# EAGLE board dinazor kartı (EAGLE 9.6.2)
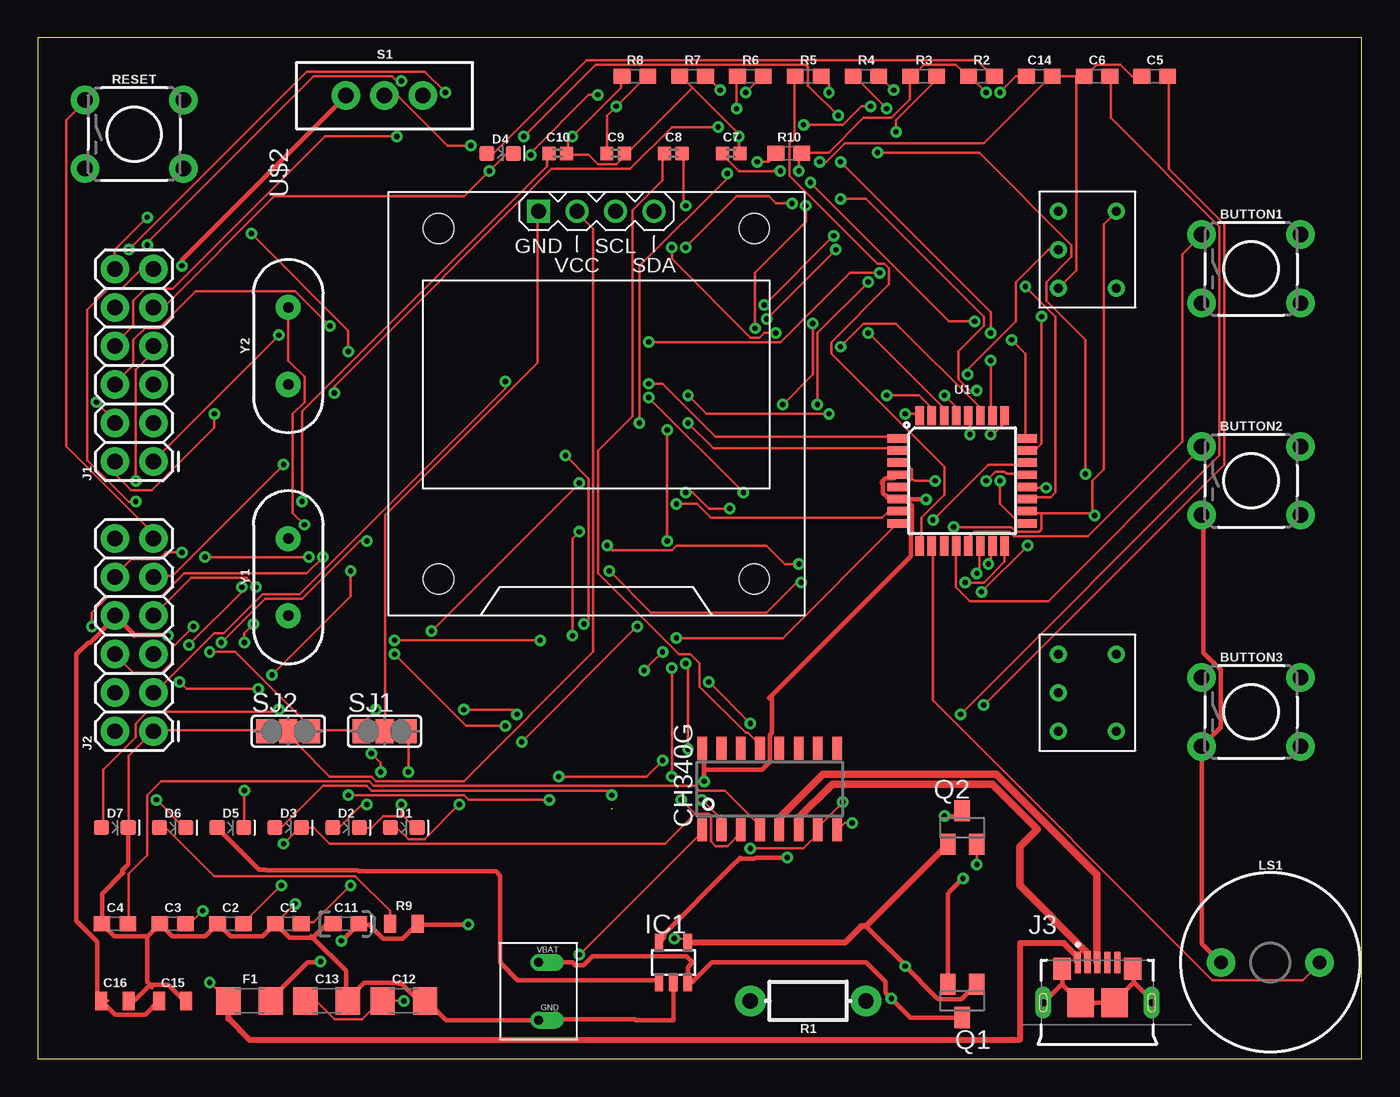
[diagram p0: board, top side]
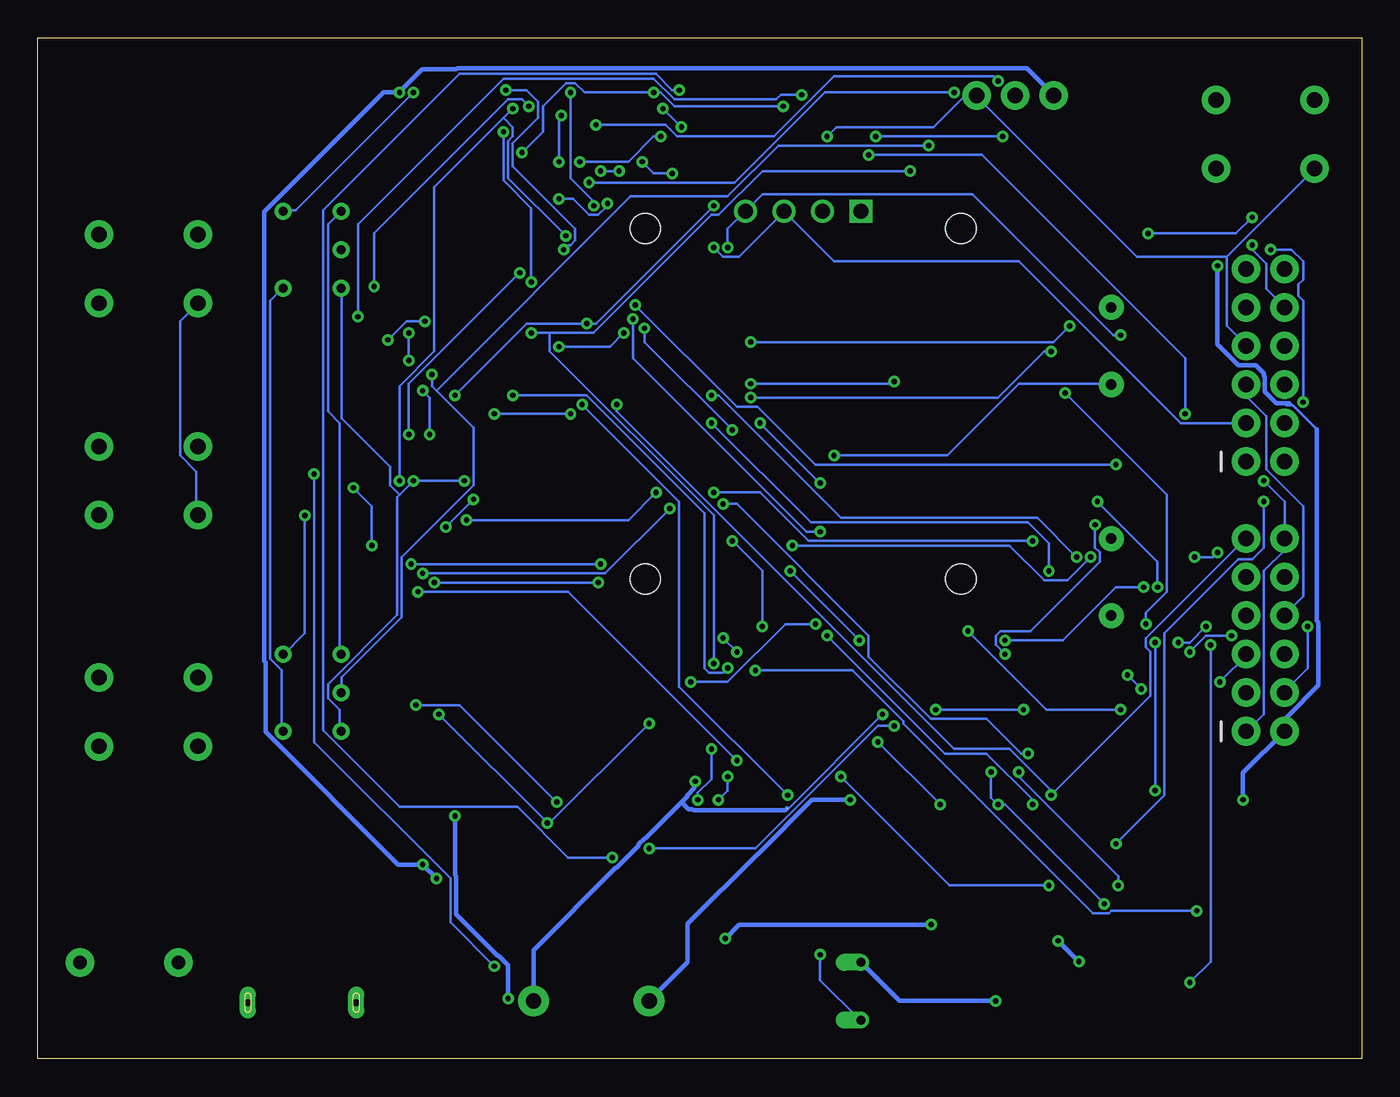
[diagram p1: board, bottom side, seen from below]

Size 87.3 x 67.3 mm. Coordinates in mm from the lower left corner, seen from the top.
Outline: 0,0 87.3,0 87.3,67.3 0,67.3 0,0
Copper layers (1*16): Top 0.035mm / dielectric 1.5mm / Bottom 0.035mm
Design rules "default": minimum track width 6mil, minimum drill 0.35mm, track to track 6mil, track to pad 6mil, pad to pad 6mil, via to via 6mil, smd to smd 6mil, copper to edge 40mil, drill to drill 6mil, minimum pad ring 10mil, minimum via ring 8mil, stop-mask expansion 4mil, vias tented up to drill 0mil, thermal gap 10mil

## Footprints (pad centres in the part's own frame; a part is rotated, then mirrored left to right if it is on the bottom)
TACTILE_SWITCH_PTH_6.0MM = drill 1.016 pad 1.88: 1 -3.251,2.261; 2 3.251,2.261; 3 -3.251,-2.261; 4 3.251,-2.261
0603 = smd 1.1 x 1: 1 -0.85,0; 2 0.85,0
0402 = smd 0.85 x 0.9: 1 -0.58,0; 2 0.58,0
0603-POLAR = smd 1.1 x 1: + 0.85,0; - -0.85,0
1206 = smd 1.6 x 1.8: 1 -1.4,0; 2 1.4,0
0805 = smd 0.8 x 1.2: 1 -0.9,0; 2 0.9,0
LED-0603 = smd 1 x 1: A -0.877,0; C 0.877,0
SOT23-5L = smd 0.55 x 1.2: 1 -0.95,-1.3; 2 0,-1.3; 3 0.95,-1.3; 4 0.95,1.3; 5 -0.95,1.3
2X6 = drill 1.016 pad 1.88: 1 0,0; 2 0,2.54; 3 2.54,0; 4 2.54,2.54; 5 5.08,0; 6 5.08,2.54; 7 7.62,0; 8 7.62,2.54; 9 10.16,0; 10 10.16,2.54; 11 12.7,0; 12 12.7,2.54
GCT_USB3075-30-A = smd 0.4 x 1.4: 1 0,0; 2 0.65,0; 3 1.3,0; 4 1.95,0; 5 2.6,0 | smd 1.15 x 1.45: S1 -1.02,-0.42; S2 3.62,-0.42 | smd 1.75 x 1.9: S3 0.175,-2.65; S4 2.425,-2.65 | drill 0.45 pad 1.05 long: S5 -2.275,-2.65; S6 4.875,-2.65
BUZZER-12MM-KIT = drill 0.9 pad 1.88: + 3.25,0; - -3.25,0
SOT23-BEC = smd 1 x 1.4: B -0.95,-1.1; C 0,1.1; E 0.95,-1.1
AXIAL-0.3-KIT = drill 1.016 pad 2.032: P$1 -3.81,0; P$2 3.81,0
SWITCH_SPDT_PTH_11.6X4.0MM = drill 1.016 pad 1.88: 1 0,2.54; 2 0,0; 3 0,-2.54
SJ_2 = smd 1.168 x 1.6: 1 -1.524,0; 2 0,0; 3 1.524,0
TQFP32-08 = smd 1.27 x 0.559: 1 -4.293,2.8; 2 -4.293,2; 3 -4.293,1.2; 4 -4.293,0.4; 5 -4.293,-0.4; 6 -4.293,-1.2; 7 -4.293,-2; 8 -4.293,-2.8; 17 4.293,-2.8; 18 4.293,-2; 19 4.293,-1.2; 20 4.293,-0.4; 21 4.293,0.4; 22 4.293,1.2; 23 4.293,2; 24 4.293,2.8 | smd 0.559 x 1.27: 9 -2.8,-4.293; 10 -2,-4.293; 11 -1.2,-4.293; 12 -0.4,-4.293; 13 0.4,-4.293; 14 1.2,-4.293; 15 2,-4.293; 16 2.8,-4.293; 25 2.8,4.293; 26 2,4.293; 27 1.2,4.293; 28 0.4,4.293; 29 -0.4,4.293; 30 -1.2,4.293; 31 -2,4.293; 32 -2.8,4.293
SOIC16 = smd 0.635 x 1.524: 1 -4.445,-2.695; 2 -3.175,-2.695; 3 -1.905,-2.695; 4 -0.635,-2.695; 5 0.635,-2.695; 6 1.905,-2.695; 7 3.175,-2.695; 8 4.445,-2.695; 9 4.445,2.695; 10 3.175,2.695; 11 1.905,2.695; 12 0.635,2.695; 13 -0.635,2.695; 14 -1.905,2.695; 15 -3.175,2.695; 16 -4.445,2.695
DISPLAY-OLED-128X64-I2C = drill 1 square: 1 -3.81,12.7 | drill 1: 2 -1.27,12.7; 3 1.27,12.7; 4 3.81,12.7 | hole 2: -10.414,11.557; 10.414,11.557; 10.414,-11.557; -10.414,-11.557
LİPOBATTERY = drill 0.6 offset: 1 -10.16,0; 2 -10.16,3.81
3.3V = drill 0.6: EN -6.35,0; GND -6.35,-2.54; IN -6.35,2.54; NC -2.54,-2.54; OUT -2.54,2.54
HC49US = drill 0.7 pad 1.651: 1 -2.54,0; 2 2.54,0

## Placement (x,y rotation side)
BUTTON1  MOMENTARY-SWITCH-SPST-PTH-6.0MM  [TACTILE_SWITCH_PTH_6.0MM]  80.01,52.07 0 top
BUTTON2  MOMENTARY-SWITCH-SPST-PTH-6.0MM  [TACTILE_SWITCH_PTH_6.0MM]  80.01,38.1 0 top
BUTTON3  MOMENTARY-SWITCH-SPST-PTH-6.0MM  [TACTILE_SWITCH_PTH_6.0MM]  80.01,22.86 0 top
C1  0.1uF  [0603]  16.51,8.89 0 top
C2  22pF  [0603]  12.7,8.89 0 top
C3  22pF  [0603]  8.89,8.89 0 top
C4  0.1uF  [0603]  5.08,8.89 0 top
C5  10pF  [0603]  73.66,64.77 0 top
C6  10pF  [0603]  69.85,64.77 0 top
C7  0.1uF  [0402]  45.72,59.69 0 top
C8  0.1uF  [0402]  41.91,59.69 0 top
C9  0.1uF  [0402]  38.1,59.69 0 top
C10  0.1uF  [0402]  34.29,59.69 0 top
C11  10uF  [0603-POLAR]  20.32,8.89 0 top
C12  4.7uF  [1206]  24.13,3.81 0 top
C13  4.7uF  [1206]  19.05,3.81 0 top
C14  0.1uF  [0603]  66.04,64.77 0 top
C15  2.2uF  [0805]  8.89,3.81 0 top
C16  10uF  [0805]  5.08,3.81 0 top
D1  BLUE  [LED-0603]  24.13,15.24 0 top
D2  BLUE  [LED-0603]  20.32,15.24 0 top
D3  GREEN  [LED-0603]  16.51,15.24 0 top
D4  Yellow  [LED-0603]  30.48,59.69 0 top
D5  GREEN  [LED-0603]  12.7,15.24 0 top
D6  GREEN  [LED-0603]  8.89,15.24 0 top
D7  RED  [LED-0603]  5.08,15.24 0 top
F1  6V/0.5A  [1206]  13.97,3.81 0 top
IC1  MCP73831  [SOT23-5L]  41.91,6.35 0 top
J1  2X6 FEMALE  [2X6]  7.62,39.37 90 top
J2  2X6 FEMALE  [2X6]  7.62,21.59 90 top
J3  USB3075-30-A  [GCT_USB3075-30-A]  68.58,6.35 0 top
LS1  BUZZER-PTH_KIT  [BUZZER-12MM-KIT]  81.28,6.35 0 top
Q1  BC327SMD  [SOT23-BEC]  60.96,3.81 180 top
Q2  BC327SMD  [SOT23-BEC]  60.96,15.24 0 top
R1  10k  [AXIAL-0.3-KIT]  50.8,3.81 180 top
R2  2.2k  [0603]  62.23,64.77 0 top
R3  2.2k  [0603]  58.42,64.77 0 top
R4  2.2k  [0603]  54.61,64.77 0 top
R5  2.2k  [0603]  50.8,64.77 0 top
R6  2.0k  [0603]  46.99,64.77 0 top
R7  2.0k  [0603]  43.18,64.77 0 top
R8  10k  [0603]  39.37,64.77 0 top
R9  0.22  [0805]  24.13,8.89 0 top
R10  2.2k  [0603]  49.53,59.69 0 top
RESET  MOMENTARY-SWITCH-SPST-PTH-6.0MM  [TACTILE_SWITCH_PTH_6.0MM]  6.35,60.96 0 top
S1  [SWITCH_SPDT_PTH_11.6X4.0MM]  22.86,63.5 270 top
SJ1  [SJ_2]  22.86,21.59 0 top
SJ2  [SJ_2]  16.51,21.59 0 top
U1  ATMEGA328P_TQFP  [TQFP32-08]  60.96,38.1 0 top
U$1  CH340G  [SOIC16]  48.26,17.78 0 top
U$2  DISPLAY-OLED-128X64-I2C  [DISPLAY-OLED-128X64-I2C]  36.83,43.18 0 top
U$3  LİPOBATTERY  [LİPOBATTERY]  43.18,2.54 0 top
U$4  3.3V  [3.3V]  73.66,53.34 0 top
U$5  3.3V  [3.3V]  73.66,24.13 0 top
Y1  16MHz  [HC49US]  16.51,31.75 90 top
Y2  16MHz  [HC49US]  16.51,46.99 90 top

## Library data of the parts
BUTTON1-BUTTON3 RESET = SparkFun-Switches; PROD_ID: SWCH-08441; SF_SKU: COM-00097
C1 C4 = SparkFun-Capacitors; PROD_ID: CAP-00810
C2 C3 = SparkFun-Capacitors; PROD_ID: CAP-07876
C5 C6 = SparkFun-Capacitors; PROD_ID: CAP-11812
C7-C10 = SparkFun-Capacitors; PROD_ID: CAP-12416
C11 = SparkFun-Capacitors; PROD_ID: CAP-13210
C12 C13 = SparkFun-Capacitors; PROD_ID: CAP-10300
C14 = SparkFun-Capacitors; PROD_ID: CAP-08604
C15 = SparkFun-Capacitors; PROD_ID: CAP-11624
C16 = SparkFun-Capacitors; PROD_ID: CAP-11330
D1 D2 = SparkFun-LED; PROD_ID: DIO-08575
D3 D5 D6 = SparkFun-LED; PROD_ID: DIO-00821
D4 = SparkFun-LED; PROD_ID: DIO-09003
D7 = SparkFun-LED; PROD_ID: DIO-00819
F1 = SparkFun-Fuses; PROD_ID: RES-08585
IC1 = microchip-update
J1 J2 = SparkFun-Connectors; PROD_ID: CONN-12423
J3 = USB3075-30-A; AVAILABILITY: In Stock; DESCRIPTION: USB - micro B USB 2.0 Receptacle Connector 5 Position Surface Mount, Right Angle; Through Hole, 2.35mm profile, 5 Pins, Horizontal, Bottom mount; MF: Global Connector Technology; MP: USB3075-30-A; PACKAGE: None; PRICE: None; PURCHASE-URL: https://pricing.snapeda.com/search/part/USB3075-30-A/?ref=eda
LS1 = SparkFun-Electromechanical; PROD_ID: COMP-08253; SF_SKU: COM-07950
Q1 Q2 = transistor-pnp
R1 = SparkFun-Resistors; PROD_ID: RES-09435
R2-R5 R10 = SparkFun-Resistors; PROD_ID: RES-08272
R6 R7 = SparkFun-Resistors; PROD_ID: RES-08296
R8 = SparkFun-Resistors; PROD_ID: RES-00824
R9 = SparkFun-Resistors; PROD_ID: RES-09883
S1 = SparkFun-Switches; PROD_ID: SWCH-08261; SF_SKU: COM-00102
SJ1 SJ2 = jumper
U1 = SparkFun-IC-Microcontroller; PROD_ID: IC-09069
U$1 = usb-serial
U$2 = diy-modules
U$3-U$5 = untitled
Y1 Y2 = SparkFun-Clocks; PROD_ID: XTAL-08181; SF_ID: COM-00536

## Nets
A0: J1.2 U1.23
A1: J1.4 U1.24
A2: J1.6 U1.25
A3: J1.8 U1.26
A4/SDA: J1.1 U1.27 U$2.4
A5/SCL: J1.3 U1.28 U$2.3
A6: J1.10 U1.19
A7: J1.12 U1.22
BUTTON1: BUTTON1.1 U1.13
BUTTON2: BUTTON2.1 U1.12
BUTTON3: U1.11
BUZZER: LS1.+ U1.10
D0/RX: D4.C J1.9 U1.30 U$1.2
D1/TX: D3.C J1.11 U1.31 U$1.3
D2: J2.4 U1.32
D3: J2.3 U1.1
D4: J2.5 U1.2
D10/SS: J2.6 U1.14
D11/MOSI: J2.10 U1.15
D12/MISO: J2.7 U1.16
D13/SCK: J2.9 R4.1 U1.17
D+: J3.3 U$1.5
D-: J3.2 U$1.6
GND: C1.1 C2.1 C3.1 C4.1 C5.1 C6.1 C7.2 C9.2 C10.2 C11.- C12.2 C13.2 C14.2 C15.2 C16.2 D1.C D2.C D7.C IC1.2 J1.7 J2.1 J2.12 R7.1 R8.1 RESET.3 S1.1 SJ1.3 SJ2.1 U1.3 U1.5 U1.21 U$1.1 U$3.1 U$4.GND U$5.GND
LED: R5.1 U1.9
N$1: D3.A R3.2
N$2: C1.2 U1.20
N$3: C4.2 U$1.4
N$4: C2.2 U1.7
N$5: C3.2 U1.8
N$6: C6.2 U$1.8 Y2.1
N$7: C5.2 U$1.7 Y2.2
N$8: D4.A R2.2
N$9: C8.1 U$1.13
N$10: SJ1.2 U$2.1
N$11: SJ2.2 U$2.2
N$12: BUTTON3.1
N$13: D2.A R4.2
N$14: D1.A R5.2
N$15: J3.S1 J3.S2 J3.S3 J3.S4 J3.S5 J3.S6
N$16: J3.5
N$17: BUTTON1.3 BUTTON2.3 BUTTON3.3 LS1.-
N$18: C10.1 F1.1 J3.1
N$19: D5.C R6.1
N$20: D5.A IC1.1
N$21: D6.A R9.1
N$22: IC1.5 R7.2
N$23: U$4.IN U$5.IN
N$24: S1.2 U$4.EN U$5.EN
N$26: U$4.NC U$5.NC
N$31: D7.A R10.1
RESET: C8.2 J2.11 R1.P$2 RESET.1 U1.29
V_BATT: C12.1 C13.1 IC1.3 Q1.C Q2.C U$3.2
VCC: C7.1 C15.1 C16.1 J1.5 J2.8 R1.P$1 R2.1 R3.1 R10.2 SJ1.1 SJ2.3 U1.4 U1.6 U1.18 U$1.16 U$4.OUT U$5.OUT
VIN: C14.1 D6.C J2.2 Q1.E Q2.E S1.3
VUSB: C9.1 C11.+ F1.2 IC1.4 Q1.B Q2.B R6.2 R8.2 R9.2

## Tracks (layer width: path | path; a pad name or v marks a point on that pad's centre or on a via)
A0  (via drill 0.35)
  Top 0.152: v66.19,48.92 66.19,40.54 65.89,40.23 65.28,40.23 U1.23 | v36.93,63.55 36.32,63.55 32.51,59.74 v32.51,59.59 | v11.63,42.52 11.63,41.6 7.52,37.49 6.15,37.49 5.08,38.56 J1.2
  Bottom 0.152: v66.19,48.92 66.19,55.02 56.59,64.62 46.69,64.62 45.31,63.25 38.61,63.25 38.3,63.55 v36.93,63.55 | v32.51,59.59 25.04,59.59 11.63,46.18 v11.63,42.52
A1  (via drill 0.35)
  Top 0.152: v64.21,47.4 65.13,46.48 65.13,41 U1.24 | v61.77,48.62 60.1,48.62 v50.95,57.76 | v26.87,63.7 25.5,65.08 17.73,65.08 v5.99,53.34 | v3.86,43.28 5.08,42.06 J1.4
  Bottom 0.152: v64.21,47.4 62.99,48.62 v61.77,48.62 | v50.95,57.76 41.35,57.76 35.41,63.7 v26.87,63.7 | v5.99,53.34 4.62,53.34 3.86,52.58 3.86,51.36 4.17,51.05 4.17,50.29 3.86,49.99 v3.86,43.28
A2  (via drill 0.35)
  Top 0.152: v62.84,41.15 62.99,41.15 63.75,41.91 63.75,42.37 U1.25 | v55.52,51.82 53.54,51.82 48.97,47.24 v40.28,47.24 | v19.25,48.31 16.97,50.6 10.41,50.6 7.98,48.16 7.06,48.16 6.3,47.4 6.3,45.72 5.08,44.5 J1.6
  Bottom 0.152: v62.84,41.15 62.84,44.5 v55.52,51.82 | v40.28,47.24 20.32,47.24 v19.25,48.31
A3  (via drill 0.35)
  Top 0.152: v62.84,46.02 62.84,42.52 U1.26 | v62.84,47.85 62.84,49.23 v52.93,59.13 | v52.78,62.18 50.8,64.16 50.8,65.38 50.65,65.53 36.78,65.53 v32.05,60.81 | v23.67,60.81 18.95,60.81 8.89,50.75 7.06,50.75 6.3,49.99 6.3,48.31 5.08,47.09 J1.8
  Bottom 0.152: v62.84,47.85 v62.84,46.02 | v52.93,59.13 52.93,62.03 v52.78,62.18 | v23.67,60.81 v32.05,60.81
A4/SDA  (via drill 0.35)
  Top 0.152: v52.93,46.94 54.46,48.46 56.59,48.46 62.08,42.98 62.08,42.52 U1.27 | v48.67,47.85 47.9,47.85 47.6,47.55 46.99,47.55 41.81,52.73 v41.81,53.49 | v15.9,47.7 7.67,39.47 J1.1
  Bottom 0.152: v52.93,46.94 49.58,46.94 v48.67,47.85 | v41.81,53.49 41.81,54.71 U$2.4 39.52,57 25.65,57 16.36,47.7 v15.9,47.7
A5/SCL  (via drill 0.35)
  Top 0.152: v61.47,41.15 61.47,42.37 U1.28 | v61.93,44.04 61.47,44.04 60.71,44.81 60.71,46.63 62.38,48.31 62.38,48.92 54.61,56.69 v52.93,56.69 | v49.73,56.39 48.67,56.39 48.21,56.84 46.08,56.84 v42.72,53.49
  Bottom 0.152: v61.47,41.15 61.47,43.59 v61.93,44.04 | v52.93,56.69 52.02,56.69 50.95,55.63 50.34,55.63 49.73,56.24 v49.73,56.39 | v42.72,53.49 42.11,52.88 41.05,52.88 38.15,55.78 U$2.3 34.8,52.58 22.61,52.58 11.94,41.91 J1.3
A6  (via drill 0.35)
  Top 0.152: v65.13,50.9 67.11,48.92 67.11,37.34 66.8,37.03 65.28,37.03 U1.19 | v54.92,62.79 54.3,62.79 53.09,61.57 v50.5,61.57 | v23.98,64.47 23.67,64.47 23.37,64.77 18.19,64.77 7.21,53.8 v7.21,53.65
  Bottom 0.152: v65.13,50.9 65.13,54.41 56.29,63.25 55.37,63.25 v54.92,62.79 | v50.5,61.57 45.92,61.57 45.16,60.81 38.76,60.81 34.8,64.77 24.28,64.77 v23.98,64.47 | v7.21,53.65 7.21,53.34 6.3,52.43 6.3,50.75 J1.10
A7  (via drill 0.35)
  Top 0.152: v59.03,35.51 62.69,39.17 65.13,39.17 U1.22 | v40.28,43.59 v46.53,37.34 | v20.47,46.63 20.47,48.01 v14.07,54.41 | v7.21,55.47 5.08,53.34 J1.12
  Bottom 0.152: v59.03,35.51 48.36,35.51 v46.53,37.34 | v40.28,43.59 23.98,43.59 20.93,46.63 v20.47,46.63 | v14.07,54.41 8.28,54.41 v7.21,55.47
BUTTON1
  Top 0.152: U1.13 61.47,33.83 61.47,34.44 61.77,34.75 64.06,34.75 64.36,34.44 69.24,34.44 75.49,40.69 75.49,53.03 76.71,54.25 BUTTON1.1
BUTTON2
  Top 0.152: U1.12 60.55,33.68 60.55,31.09 61.47,30.18 66.65,30.18 76.71,40.23 BUTTON2.1
BUZZER
  Top 0.152: U1.10 59.03,33.68 59.03,23.62 77.47,5.18 83.41,5.18 84.48,6.25 LS1.+
D0/RX  (via drill 0.35)
  Top 0.152: J1.9 8.28,49.53 15.6,56.84 28.09,56.84 v29.77,58.52 30.84,59.59 31.29,59.59 D4.C | v54.76,47.85 59.64,42.98 59.64,42.52 U1.30 | v43.79,17.07 45.01,15.85 45.01,15.09 U$1.2 | v42.88,20.42 42.88,25.91 v42.72,26.06
  Bottom 0.152: 53.54,47.85 50.65,47.85 42.88,55.63 42.42,55.63 39.52,58.52 v29.77,58.52 | 53.54,47.85 v54.76,47.85 | v43.79,17.07 43.79,17.53 42.88,18.44 v42.88,20.42 | v42.72,26.06 42.72,35.81 53.54,46.63 53.54,47.85
D1/TX  (via drill 0.35)
  Top 0.152: 43.33,16.15 41.35,14.17 19.25,14.17 18.19,15.24 D3.C 17.27,15.24 v16.21,14.17 | 43.33,16.15 44.25,16.15 44.4,16 44.4,14.33 44.7,14.02 45.47,14.02 46.38,14.94 U$1.3 | v55.98,43.74 58.12,43.74 58.88,42.98 58.88,42.52 U1.31 | v41.81,18.59 v41.81,25.76 | 43.33,16.15 v42.42,17.07 | v6.45,36.73 5.99,36.73 3.25,39.47 3.25,49.38 4.62,50.75 5.54,50.75 6.76,51.97 7.52,51.97 J1.11
  Bottom 0.152: v55.98,43.74 51.11,43.74 43.33,35.97 43.33,25.76 43.03,25.45 42.11,25.45 v41.81,25.76 | v41.81,18.59 41.81,17.68 v42.42,17.07 | v6.45,36.73 6.45,33.68 7.21,32.92 8.13,32.92 13,28.04 13,17.37 v16.21,14.17
D2  (via drill 0.35)
  Top 0.152: v57.2,42.52 58.12,42.52 U1.32 | v52.17,42.52 44.09,42.52 v42.88,43.74 | v18.8,33.07 17.73,32 9.65,32 8.13,30.48 4.62,30.48 3.56,29.41 v3.56,28.5
  Bottom 0.152: v52.17,42.52 v57.2,42.52 | v42.88,43.74 42.42,43.74 34.34,35.66 21.39,35.66 v18.8,33.07 | v3.56,28.5 3.56,25.76 5.08,24.23 J2.4
D3  (via drill 0.35)
  Top 0.152: v40.28,44.5 41.2,44.5 44.7,41 56.59,41 U1.1 | v30.84,44.65 30.84,44.2 17.27,30.63 14.83,30.63 12.24,28.04 11.63,28.04 7.67,24.08 J2.3
  Bottom 0.152: v40.28,44.5 30.99,44.5 v30.84,44.65
D4  (via drill 0.35)
  Top 0.152: v42.88,41.91 44.55,40.23 56.59,40.23 U1.2 | v20.62,32.16 20.62,30.48 v15.44,25.3 | v14.53,24.38 9.8,24.38 v9.35,24.84
  Bottom 0.152: v42.88,41.91 36.32,35.36 22,35.36 20.62,33.98 v20.62,32.16 | v14.53,24.38 v15.44,25.3 | v9.35,24.84 7.52,26.67 J2.5
D10/SS  (via drill 0.35)
  Top 0.152: v61.93,32 62.08,32.16 62.08,33.68 U1.14 | v45.62,36.27 44.25,36.27 43.18,37.34 v42.72,37.34 | v21.69,34.14 21.23,34.14 17.42,30.33 14.99,30.33 v12.09,27.43 | v10.26,28.5 8.89,27.13 8.89,26.21 8.13,25.45 6.3,25.45 J2.6
  Bottom 0.152: v61.93,32 49.89,32 v45.62,36.27 | v42.72,37.34 39.68,37.34 36.47,34.14 v21.69,34.14 | v12.09,27.43 11.33,27.43 v10.26,28.5
D11/MOSI  (via drill 0.35)
  Top 0.152: v62.69,32.61 62.84,32.77 62.84,33.68 U1.15 | v50.19,32.61 49.28,32.61 48.06,33.83 42.11,33.83 41.81,33.53 37.85,33.53 v37.54,33.83 | v11.02,33.07 v17.88,33.07 | v9.5,33.38 8.43,33.38 7.98,32.92 6.15,32.92 5.08,31.85 J2.10
  Bottom 0.152: v50.19,32.61 v62.69,32.61 | v37.54,33.83 23.22,33.83 20.93,31.55 19.41,31.55 v17.88,33.07 | v11.02,33.07 9.8,33.07 v9.5,33.38
D12/MISO  (via drill 0.35)
  Top 0.152: v61.16,31.39 62.38,31.39 63.75,32.77 63.75,33.68 U1.16 | v50.34,31.39 50.04,31.39 48.06,29.41 40.44,29.41 v37.69,32.16 | v23.52,27.58 v33.12,27.58 | v14.38,31.09 13.77,31.7 10.11,31.7 J2.7
  Bottom 0.152: v50.34,31.39 v61.16,31.39 | v33.12,27.58 v37.69,32.16 | v23.52,27.58 19.71,27.58 16.21,31.09 v14.38,31.09
D13/SCK  (via drill 0.35)
  Top 0.152: v55.98,62.64 53.85,64.77 R4.1 | v63.45,38.1 63.45,36.58 64.67,35.36 65.13,35.36 U1.17 | v16.21,39.17 8.89,31.85 7.67,31.85 J2.9 | v52.48,54.25 v47.9,49.68
  Bottom 0.152: 56.59,62.03 61.16,57.45 61.16,46.63 63.45,44.35 v63.45,38.1 | 56.59,62.03 v55.98,62.64 | v16.21,39.17 36.02,39.17 39.83,42.98 41.2,42.98 v47.9,49.68 | v52.48,54.25 56.29,58.06 56.29,60.5 55.98,60.81 55.98,61.42 56.59,62.03
D+
  Top 0.152: 48.97,15.39 48.97,15.24 48.97,15.09 U$1.5 | 69.85,6.4 J3.3
  Top 0.508: J3.3 69.85,6.38 69.85,12.12 63.21,18.76 51.78,18.76 51.03,18.01 50.8,17.78 48.97,15.95 48.97,15.24
D-
  Top 0.152: 50.19,15.39 50.19,15.09 U$1.6 | 69.09,6.4 J3.2
  Top 0.508: J3.2 69.23,6.97 64.77,11.43 64.77,13.97 65.92,15.12 62.94,18.1 52.39,18.1 50.17,15.88 U$1.6
GND  (via drill 0.35)
  Top 0.152: SJ2.1 14.99,21.64 7.67,21.64 J2.1 5.99,19.96 5.99,15.24 D7.C 5.84,15.24 | 41.81,4.57 41.81,5.03 IC1.2 | 39.83,2.59 39.37,2.59 | 33.12,2.59 U$3.1 32.97,2.59 | v35.71,6.86 43.79,14.94 U$1.1 | 4.32,8.84 C4.1 4.32,8.99 | 7.98,8.84 C3.1 8.13,8.84 | 6.35,3.81 C16.2 | D2.C 22,15.24 22.76,16 23.98,16 | 23.98,16 24.13,16 24.89,15.24 D1.C | v24.43,18.9 24.43,21.49 SJ1.3 | 23.98,16 v23.98,16.76 | 11.94,8.84 C2.1 11.79,8.84 | 15.6,8.84 C1.1 | 19.05,8.84 19.41,8.84 C11.- | 15.75,8.84 C1.1 | 20.32,3.81 C13.2 20.47,3.81 | 25.04,3.81 25.4,3.81 C12.2 25.65,3.81 | 21.67,5 21.69,5.03 | v16.97,10.21 15.75,8.99 C1.1 | 26.8,2.67 26.87,2.59 | C6.1 68.48,64.77 | 68.48,64.77 C14.2 66.8,64.77 62.38,60.35 53.24,60.35 52.02,59.13 v51.56,59.13 | C5.1 72.14,64.77 71.37,65.53 69.85,65.53 69.09,64.77 C6.1 | 57.66,38.25 57.2,37.8 56.74,37.8 U1.5 | 57.66,38.25 57.66,38.86 57.35,39.17 56.74,39.17 U1.3 | v62.54,38.1 63.14,38.71 63.75,38.71 63.91,38.56 65.13,38.56 U1.21 | v59.18,38.1 57.81,38.1 57.66,38.25 | 68.48,64.77 68.48,51.97 U$4.GND | 68.94,64.77 C6.1 | 43.18,64.01 42.42,64.77 R7.1 | 43.18,64.01 46.23,60.96 v46.23,60.81 46.23,59.74 C7.2 | 38.76,59.59 38.15,58.98 36.93,58.98 36.32,59.59 34.95,59.59 C10.2 34.95,59.74 34.95,60.5 v35.26,60.81 38.46,64.01 38.46,64.77 R8.1 | 38.76,59.59 43.18,64.01 | 38.76,59.59 C9.2 | v6.45,38.1 6.45,45.41 7.52,46.48 7.52,46.94 J1.7
  Top 0.305: IC1.2 41.91,2.54 39.42,2.54 39.37,2.59 32.97,2.59 | U$3.1 26.92,2.54 26.8,2.67 25.65,3.81 25.4,3.81 | C12.2 25.1,3.81 23.98,4.93 | 23.82,5.03 23.88,5.03 23.98,4.93 | 23.98,4.93 23.74,4.93 23.66,5.01 21.8,5.01 21.79,5 21.67,5 21.51,5 20.32,3.81 | C13.2 20.32,3.94 20.32,5.79 18.14,7.98 | 18.03,8.08 18.14,7.98 | 18.14,7.98 19,8.84 19.05,8.84 | 18.14,7.98 16.61,7.98 15.75,8.84 | 15.6,8.84 14.83,8.08 12.7,8.08 11.94,8.84 | C2.1 11.04,8.08 8.85,8.08 C3.1 7.23,8.08 7.21,8.08 | 7.21,5.03 7.21,5.08 | 7.21,5.08 7.21,8.08 | 7.21,8.08 5.04,8.08 C4.1 4.23,10.88 5.56,12.22 | 5.56,12.22 5.61,12.27 | 5.56,12.22 5.56,12.42 5.96,12.81 D7.C | 7.21,5.08 7.42,4.88 | 7.42,4.88 7.52,4.78 | 7.52,4.78 7.52,4.72 | 7.42,4.88 8.59,4.88 9.65,3.81 C15.2 | 6.35,3.81 7.31,4.78 7.52,4.78
  Bottom 0.152: J2.1 7.52,21.64 6.45,22.71 6.45,32.16 5.08,33.53 J2.12 5.08,36.73 v6.45,38.1 | v35.71,6.86 35.71,5.18 33.12,2.59 U$3.1 | v24.43,18.9 24.43,17.22 v23.98,16.76 23.52,16.76 v16.97,10.21 | v59.18,38.1 v62.54,38.1 63.45,37.19 | 63.45,37.19 63.6,37.03 63.6,29.26 68.17,24.69 68.17,23.77 67.41,23.01 67.41,21.64 U$5.GND | 63.45,37.19 64.06,37.8 64.06,39.01 67.26,42.22 67.26,50.75 U$4.GND | 8.89,52.88 3.1,58.67 RESET.3 | 8.89,52.88 8.89,48.31 7.67,47.09 J1.7 | v35.26,60.81 34.65,61.42 28.25,61.42 26.26,63.4 25.5,63.4 S1.1 25.35,63.4 14.83,52.88 8.89,52.88 | v51.56,59.13 48.36,59.13 46.69,60.81 v46.23,60.81
LED
  Top 0.152: R5.1 49.89,64.77 49.89,60.66 49.58,60.35 49.58,58.22 55.37,52.43 55.83,52.43 56.13,52.12 56.13,51.05 52.32,47.24 52.32,46.48 59.79,39.01 59.79,37.19 58.27,35.66 58.27,33.83 U1.9
N$1  (via drill 0.35)
  Top 0.152: D3.A 16.05,15.24 18.8,17.98 21.69,17.98 22,17.68 37.54,17.68 v37.85,17.37 | v51.41,43.13 51.41,47.85 v54.76,51.21 | v56.59,61.11 56.59,61.87 59.18,64.47 59.18,64.77 R3.2
  Bottom 0.152: v37.85,17.37 45.01,24.54 45.01,36.73 v51.41,43.13 | v54.76,51.21 54.76,56.08 56.59,57.91 v56.59,61.11
N$2  (via drill 0.35)
  Top 0.152: v20.62,11.43 18.19,8.99 17.42,8.99 C1.2 | v34.34,18.59 40.13,18.59 v41.2,19.66 | v65.28,33.83 v62.23,30.79 | v66.5,37.64 65.28,37.64 U1.20
  Bottom 0.152: v20.62,11.43 27.18,11.43 v34.34,18.59 | v41.2,19.66 52.32,30.79 v62.23,30.79 | v65.28,33.83 65.28,36.42 v66.5,37.64
N$3
  Top 0.152: C4.2 5.99,8.99 5.99,12.19 7.21,13.41 7.21,17.37 8.13,18.29 21.84,18.29 22.15,17.98 43.33,17.98 43.64,17.68 45.31,17.68 47.6,15.39 47.6,15.09 U$1.4
N$4  (via drill 0.35)
  Top 0.152: v16.05,11.43 13.61,8.99 C2.2 | v22.61,18.9 22.61,19.51 v22,20.12 | v42.11,36.58 43.49,36.58 44.4,35.66 55.68,35.66 55.98,35.97 56.59,35.97 U1.7
  Bottom 0.152: v16.05,11.43 16.05,12.04 22.61,18.59 v22.61,18.9 | v22,20.12 22.45,20.12 24.74,22.4 28.4,22.4 32.51,26.52 32.51,27.89 41.2,36.58 v42.11,36.58
N$5  (via drill 0.35)
  Top 0.152: v10.87,9.75 10.11,8.99 9.8,8.99 C3.2 | v41.2,26.82 v39.98,25.6 | v42.11,27.74 49.12,27.74 56.59,35.2 U1.8
  Bottom 0.152: v10.87,9.75 16.51,9.75 16.66,9.6 17.73,9.6 30.23,22.1 30.23,22.25 33.58,25.6 v39.98,25.6 | v42.11,27.74 v41.2,26.82
N$6  (via drill 0.35)
  Top 0.152: v60.86,22.71 77.93,39.78 77.93,54.86 70.76,62.03 70.76,64.77 C6.2 | v53.7,15.54 53.24,15.54 52.78,15.09 U$1.8 | v34.8,39.78 36.32,38.25 36.32,28.96 v36.02,28.65 | v46.99,22.1 v44.25,24.84
  Bottom 0.152: v60.86,22.71 v53.7,15.54 53.54,15.54 v46.99,22.1 | v34.8,39.78 27.33,39.78 22.61,44.5 16.51,44.5 Y2.1 | v36.02,28.65 38,28.65 41.81,24.84 v44.25,24.84
N$7  (via drill 0.35)
  Top 0.152: v62.38,23.32 78.23,39.17 78.23,55.02 74.57,58.67 74.57,64.77 C5.2 | v53.09,16.92 51.56,15.39 51.56,15.09 U$1.7 51.56,14.94 50.5,13.87 v46.99,13.87 | Y2.2 16.51,46.02 17.58,44.96 17.58,43.28 16.82,42.52 16.82,35.97 v17.58,35.2 | v23.52,26.67 28.25,21.95 v30.84,21.95
  Bottom 0.152: v62.38,23.32 59.49,23.32 v53.09,16.92 | v17.58,35.2 17.58,33.68 17.27,33.38 17.27,32.77 21.84,28.19 23.82,28.19 24.13,27.89 24.13,27.28 v23.52,26.67 | v30.84,21.95 31.9,21.95 39.98,13.87 v46.99,13.87
N$8
  Top 0.152: D4.A 29.62,59.74 30.07,59.74 36.17,65.84 61.93,65.84 62.99,64.77 R2.2
N$9
  Top 0.152: C8.1 41.2,59.59 41.2,57.91 39.22,55.93 39.22,42.37 36.93,40.08 36.93,32 42.27,26.67 43.03,26.67 43.64,26.06 43.64,24.54 46.69,21.49 46.84,21.49 47.75,20.57 U$1.13
N$10
  Top 0.152: SJ1.2 22.91,21.64 22.91,35.81 32.97,45.87 32.97,55.78 U$2.1
N$11
  Top 0.152: SJ2.2 16.51,21.49 17.12,20.88 17.12,20.73 19.25,18.59 22,18.59 22.3,18.29 28.09,18.29 36.63,26.82 36.63,54.71 35.56,55.78 U$2.2
N$13  (via drill 0.35)
  Top 0.152: D2.A 19.86,15.24 21.39,16.76 v21.69,16.76 | v35.26,27.89 35.26,34.29 v35.71,34.75 | v52.63,53.34 v48.06,48.77 | v56.44,63.86 55.52,64.77 R4.2
  Bottom 0.152: v21.69,16.76 21.69,17.07 24.74,20.12 27.48,20.12 v35.26,27.89 | v35.71,34.75 36.63,34.75 48.06,46.18 v48.06,48.77 | v52.63,53.34 52.32,53.65 52.17,53.65 51.87,53.95 51.87,54.71 55.98,58.83 55.98,60.35 54.3,62.03 54.3,63.09 55.07,63.86 v56.44,63.86
N$14  (via drill 0.35)
  Top 0.152: D1.A 23.67,15.24 24.43,14.48 25.5,14.48 v27.79,16.76 | v39.52,28.5 v31.9,20.88 | v41.5,41.45 v41.5,34.14 | v47.3,48.16 47.3,51.82 50.65,55.17 v50.65,56.24 | v52.17,63.7 52.17,64.31 51.71,64.77 R5.2
  Bottom 0.152: v31.9,20.88 v27.79,16.76 | v39.52,28.5 39.52,32.16 v41.5,34.14 | v41.5,41.45 47.3,47.24 v47.3,48.16 | v50.65,56.24 50.65,56.54 52.17,58.06 v52.17,63.7
N$15
  Top 0.152: 67.56,4.88 67.56,5.03 | 67.56,5.79 J3.S1 | 68.63,3.81 J3.S3 68.78,3.66 | 72.29,5.79 J3.S2 | 73.35,3.81 J3.S6 | 71.07,3.81 J3.S4 70.92,3.66
  Top 0.305: 72.29,5.03 73.45,3.86 J3.S6 | 72.29,5.03 72.29,5.79 | 72.29,5.03 71.12,3.86 71.12,3.81 71.07,3.81 | J3.S4 J3.S3 67.56,4.89 | 67.56,4.89 67.56,5.03 67.56,5.79 | 67.56,4.89 67.5,4.89 J3.S5
N$17
  Top 0.152: 76.86,20.57 BUTTON3.3 76.86,20.73 | 77.93,6.4 LS1.- | 76.86,35.81 BUTTON2.3
  Top 0.305: 77.93,6.4 76.76,7.57 BUTTON3.3 76.76,20.62 78,21.87 78,25.64 | 77.93,25.76 78,25.68 78,25.64 | 78,25.64 76.86,26.78 76.86,26.82 76.86,35.81
  Bottom 0.152: BUTTON2.3 76.86,35.97 76.86,38.71 77.93,39.78 77.93,48.62 76.86,49.68 BUTTON1.3
N$18  (via drill 0.35)
  Top 0.152: v17.42,36.73 17.42,42.67 33.58,58.83 33.58,59.59 C10.1 | v13.46,31.09 13.46,30.79 v9.96,27.28 | v11.33,5.03 12.55,3.81 F1.1 12.7,3.81 | 68.48,6.71 68.48,6.4 J3.1
  Top 0.406: J3.1 68.49,6.44 68.49,6.8 67.67,7.62 64.77,7.62 64.77,1.27 64.72,1.22 13.97,1.22 12.57,2.62 F1.1
  Bottom 0.152: v17.42,36.73 13.46,32.77 v13.46,31.09 | v9.96,27.28 9.96,6.4 v11.33,5.03
N$19  (via drill 0.35)
  Top 0.152: v13.61,17.68 13.61,15.24 D5.C | v13.61,27.43 13.61,28.04 v14.22,28.65 | v19.56,43.89 19.56,44.35 33.88,58.67 39.07,58.67 41.81,61.42 v44.86,61.42 | v46.08,62.64 46.08,64.77 R6.1
  Bottom 0.152: v13.61,27.43 v13.61,17.68 | v14.22,28.65 14.22,29.41 12.85,30.79 12.85,37.19 v19.56,43.89 | v46.08,62.64 v44.86,61.42
N$20
  Top 0.152: 12.24,15.24 D5.A | 15.14,12.34 15.01,12.47 | 25.81,12.34 25.4,12.34 | 40.89,5.18 IC1.1
  Top 0.305: IC1.1 40.83,5.18 31.65,5.18 30.48,6.35 30.48,12.06 30.2,12.34 25.4,12.34 21.16,12.34 21.09,12.42 15.06,12.42 15.01,12.47 14.59,12.47 D5.A
N$21
  Top 0.152: D6.A 8.43,15.24 11.63,12.04 20.93,12.04 23.22,9.75 23.22,8.99 R9.1
N$22  (via drill 0.35)
  Top 0.152: v45.01,63.86 44.09,64.77 R7.2 | 40.89,7.77 IC1.5
  Top 0.305: IC1.5 41.28,7.97 41.28,8.21 45.75,12.68 46.26,13.19 | 46.26,13.19 46.33,13.26 | v49.43,13.26 47.35,13.26 47.27,13.19 46.26,13.19
  Bottom 0.152: v45.01,63.86 45.47,63.86 46.53,64.92 59.49,64.92 68.48,55.93 68.48,21.64 63.45,16.61 55.68,16.61 52.32,13.26 v49.43,13.26
N$23
  Bottom 0.152: U$4.IN 68.17,55.02 68.17,42.67 67.41,41.91 67.41,26.67 U$5.IN
N$24  (via drill 0.35)
  Top 0.152: v61.32,45.11 61.32,45.41 64.52,48.62 64.52,51.21 66.65,53.34 U$4.EN | v28.55,60.2 27.03,60.2 23.82,63.4 22.91,63.4 S1.2
  Bottom 0.152: 61.01,44.04 61.32,44.35 v61.32,45.11 | 61.01,44.04 58.57,41.6 58.57,37.8 63.3,33.07 63.3,29.11 67.26,25.15 67.26,24.23 U$5.EN | v28.55,60.2 38.46,60.2 41.81,56.84 48.21,56.84 61.01,44.04
N$26
  Bottom 0.152: U$5.NC 71.22,21.64 71.22,25.6 71.98,26.36 71.98,49.99 71.22,50.75 U$4.NC
N$31  (via drill 0.35)
  Top 0.152: v15.9,23.01 15.75,22.86 7.21,22.86 6.45,22.1 6.45,21.18 4.32,19.05 4.32,15.24 D7.A | v35.71,37.95 v25.96,28.19 | v39.68,41.91 39.68,52.27 45.47,58.06 v45.47,58.37 | v47.45,59.13 48.21,59.13 48.67,59.59 R10.1
  Bottom 0.152: v15.9,23.01 20.78,23.01 v25.96,28.19 | v39.68,41.91 v35.71,37.95 | v45.47,58.37 46.69,58.37 v47.45,59.13
RESET  (via drill 0.35)
  Top 0.152: v42.72,56.24 42.57,56.39 42.57,59.59 C8.2 | v59.79,43.74 60.55,42.98 60.55,42.52 U1.29 | J2.11 7.52,34.29 7.52,34.75 1.88,40.39 1.88,61.87 3.1,63.09 RESET.1 | v33.73,17.07 28.4,17.07 28.09,17.37 v20.47,17.37 | v51.11,48.46 51.11,45.11 v49.12,43.13
  Bottom 0.152: v42.72,56.24 50.5,48.46 v51.11,48.46 55.07,48.46 v59.79,43.74 | 20.32,17.53 13.92,23.93 13.92,26.82 14.22,27.13 14.22,27.74 7.67,34.29 J2.11 | v49.12,43.13 49.12,42.67 26.87,20.42 23.22,20.42 20.32,17.53 | 20.32,17.53 v20.47,17.37
  Bottom 0.305: R1.P$2 44.45,6.35 44.45,8.89 39.85,13.49 39.82,13.49 36.24,17.07 v33.73,17.07
V_BATT  (via drill 0.35)
  Top 0.152: C13.1 18.34,3.81 19.56,2.59 21.39,2.59 22.61,3.81 C12.1 v24.13,3.81 | 42.72,5.49 42.72,5.18 IC1.3 42.88,5.18 | 33.12,6.25 U$3.2 | 56.16,4.09 v56.29,3.96 | 60.86,2.74 Q1.C | Q2.C 60.86,16.31
  Top 0.305: Q1.C 57.54,2.71 56.16,4.09 | v56.29,3.96 55.93,4.32 55.93,4.36 55.88,4.41 55.88,5.08 54.61,6.35 44.45,6.35 43.15,5.05 IC1.3 42.86,6.03 43.18,6.35 42.79,6.75 36.57,6.75 36,6.17 35.43,6.17 35.25,6.35 U$3.2 | 60.86,16.31 60.55,16 v59.79,16
  Bottom 0.152: 59.79,9.6 59.39,9.2 | 30.53,3.81 30.48,3.81 | 32.97,6.25 U$3.2
  Bottom 0.305: U$3.2 30.48,3.81 v24.13,3.81 | v59.79,16 59.79,12.12 59.72,12.04 59.72,9.53 59.39,9.2 56.97,6.78 56.92,6.78 56.29,6.15 56.29,6.1 v56.29,3.96
VCC  (via drill 0.35)  (1 unrouted)
  Top 0.152: 18.03,21.64 21.23,21.64 SJ1.1 21.39,21.64 21.39,22.1 v22.3,23.01 | 4.62,3.81 C16.1 4.17,3.81 | 7.98,3.81 C15.1 | 18.03,21.64 17.42,22.25 17.42,22.4 13,26.82 v11.33,26.82 | 6.3,27.89 6.35,27.89 | 18.03,21.64 SJ2.3 | 43.94,20.42 U$1.16 | 55.68,37.34 55.98,37.03 | 56.13,38.41 56.59,38.41 U1.4 | 69.55,35.97 66.19,35.97 | 66.19,35.97 65.28,35.97 U1.18 | v60.4,35.05 64.21,35.05 64.52,34.75 66.04,34.75 66.19,34.9 66.19,35.97 | 56.74,36.88 U1.6 | v48.97,58.52 46.23,58.52 45.16,59.59 C7.1 | v50.19,58.52 50.19,59.44 50.34,59.59 R10.2 50.5,59.74 52.17,59.74 54.46,62.03 56.29,62.03 57.51,63.25 57.51,64.77 R3.1 57.66,64.77 58.42,65.53 60.55,65.53 61.32,64.77 R2.1 61.47,64.77 v62.54,63.7 | 69.55,35.97 69.55,38.1 70.31,38.86 70.31,55.02 71.07,55.78 U$4.OUT | 69.55,35.97 v69.7,35.81 | 48.21,19.51 48.06,19.36 | v28.09,23.01 31.29,23.01 v31.6,22.71
  Top 0.305: U1.4 56.45,38.28 55.91,38.28 55.68,38.05 | 55.68,37.95 55.68,38.05 | 55.68,38.05 55.73,38 55.73,37.29 55.98,37.04 55.98,37.03 56.53,37.03 U1.6 57.15,36.9 | 57.15,36.9 58.55,36.9 v58.57,36.88 | 57.15,36.9 57.37,36.68 57.43,36.68 57.66,36.45 57.66,34.65 57.58,34.57 57.58,33.14 48.41,23.98 | 48.21,23.77 48.41,23.98 | 48.41,23.98 48.41,21.5 48.27,21.36 48.27,19.57 48.06,19.36 47.75,19.05 43.94,19.05 | 43.94,19.05 43.94,20.35 U$1.16 | 43.94,19.05 v43.94,18.29 | 7.98,3.81 7.06,2.9 5.09,2.9 C16.1 3.91,4.08 3.91,7.72 2.54,9.09 2.54,26.67 3.3,27.43 3.46,27.43 5.08,29.06 J2.8 6.35,27.94 | 6.35,27.89 6.35,27.94 | 6.35,27.94 8.53,27.94 v8.59,27.89
  Bottom 0.152: v11.33,26.82 10.26,27.89 v8.59,27.89 | J1.5 7.52,44.35 7.52,43.59 6.3,42.37 6.3,38.86 3.86,36.42 3.86,30.48 5.08,29.26 J2.8 | v69.7,35.81 69.7,28.04 71.07,26.67 U$5.OUT | v60.4,35.05 v58.57,36.88 | v50.19,58.52 v48.97,58.52 | v62.54,63.7 70.31,55.93 71.07,55.93 U$4.OUT | v28.09,23.01 v22.3,23.01 | 37.85,16.46 v31.6,22.71
  Bottom 0.305: R1.P$1 54.61,7.16 49.2,12.58 49.15,12.58 47.67,14.05 47.67,14.15 47.27,14.55 47.22,14.55 44.86,16.92 | 44.86,16.92 44.47,17.3 44.47,17.38 43.98,17.87 43.98,18.25 v43.94,18.29 | 44.86,16.92 44.4,16.46 44.15,16.46 44.07,16.39 38,16.39 37.89,16.5
VIN  (via drill 0.35)
  Top 0.152: v7.82,17.07 9.65,15.24 D6.C | 60.12,11 60.1,10.97 | v61.93,12.8 61.93,14.02 Q2.E | 60.1,5.03 Q1.E | C14.1 64.52,64.77 v63.45,63.7 | 9.5,52.58 v9.5,52.27 | 20.32,63.4 S1.3
  Top 0.305: Q1.E 60.01,10.89 60.12,11 v61.01,11.89 | S1.3 9.5,52.68 v9.5,52.27
  Bottom 0.152: 5.08,21.49 J2.2 5.08,22.4
  Bottom 0.203: 5.08,43.2 4.98,43.1 4.59,43.1 2.97,41.48 2.95,41.47 2.95,41.45
  Bottom 0.305: v61.01,11.89 v61.93,12.8 | v61.93,12.8 62.23,12.8 | v61.93,12.8 63.55,12.8 72.29,21.54 72.29,26.13 72.36,26.21 72.36,55.85 64.52,63.7 v63.45,63.7 63.22,63.94 63.22,63.99 61.98,65.23 59.72,65.23 59.65,65.3 22.07,65.3 20.32,63.55 S1.3 | v9.5,52.27 9.5,47.09 8.13,45.72 6.98,45.72 6.45,45.19 6.45,45.04 6.38,44.97 6.38,43.97 5.61,43.2 5.08,43.2 4.78,43.2 | 2.97,41.48 2.97,28.88 2.87,28.78 2.87,24.61 3.83,23.65 3.83,23.61 5.08,22.37 J2.2 7.82,18.85 7.82,18.75 v7.82,17.07
VUSB  (via drill 0.35)
  Top 0.152: 21.59,8.84 21.23,8.84 C11.+ 21.08,8.84 | 24.89,8.84 R9.2 25.04,8.84 | 15.44,3.81 F1.2 | C9.1 37.54,59.74 37.54,62.18 v38.15,62.79 40.13,64.77 R8.2 | v46.69,63.7 47.75,64.77 R6.2 | 42.88,7.77 IC1.4 42.72,7.77 42.57,7.92 v41.96,7.92 | 59.94,14.02 Q2.B | 61.77,4.88 Q1.B | v55.37,59.74 62.08,59.74 68.17,53.65 68.17,52.88 66.5,51.21 66.5,49.99 69.09,47.4 v69.09,38.56
  Top 0.305: 54.61,8.69 54.61,8.74 57.2,6.15 v57.2,6.1 59.21,4.09 59.21,4.08 59.38,3.9 60.91,3.9 Q1.B | v28.4,8.84 25.08,8.84 R9.2 24.07,7.92 22.76,7.92 21.84,8.84 21.59,8.84 | C11.+ 20.05,7.77 v20.02,7.77 | v18.64,6.4 18.59,6.35 17.78,6.35 15.37,3.94 F1.2
  Top 0.406: Q2.B 54.61,8.74 54.31,8.74 53.23,7.66 IC1.4
  Bottom 0.152: v38.15,62.79 45.31,62.79 46.23,63.7 v46.69,63.7 51.26,63.7 51.87,64.31 52.48,64.31 54,62.79 54,61.11 v55.37,59.74 | v69.09,38.56 69.09,20.88 60.1,11.89 60.1,8.99 v57.2,6.1
  Bottom 0.305: v41.96,7.92 41.05,8.84 v28.4,8.84 | v20.02,7.77 v18.64,6.4

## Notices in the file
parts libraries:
SparkFun-Switches: Licensing: Creative Commons ShareAlike 4.0 International - https://creativecommons.org/licenses/by-sa/4.0
diy-modules: Released under the Creative Commons Attribution 4.0 International License: http://creativecommons.org/licenses/by/4.0
